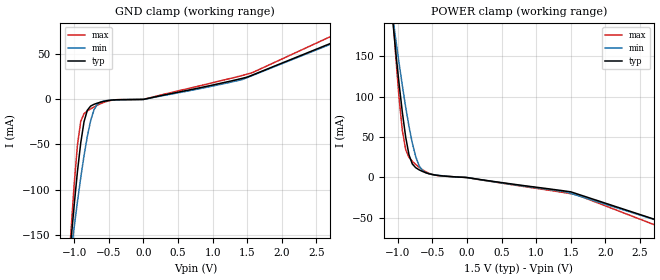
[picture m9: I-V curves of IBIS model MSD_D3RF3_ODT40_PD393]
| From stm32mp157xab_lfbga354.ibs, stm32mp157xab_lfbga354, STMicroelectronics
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[Model] MSD_D3RF3_ODT40_PD393
Model_type   Input
C_comp 2.254pF   2.214pF   2.330pF
Vinh = 925.000mV
Vinl = 575.000mV
[Model Spec]
Vinh   925.000mV   888.000mV   963.000mV
Vinl   575.000mV   538.000mV   613.000mV
[Temperature Range]   25.000   125.000   -40.000
[Voltage Range]   1.500V   1.425V   1.575V
[GND Clamp Reference]   0.00V   0.00V   0.00V
[POWER Clamp Reference]   1.500V   1.425V   1.575V
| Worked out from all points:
|   GND clamp passes 1 mA (typ) near -0.49 V on its own axis
|   POWER clamp passes 1 mA (typ) near -0.21 V on its own axis
[GND Clamp]
-1.48V    -589mA     -456.8mA   -787.9mA
-1.05V    -159mA     -171.5mA   -149.1mA
-1.002V   -117.6mA   -142mA     -94.67mA
-954.6mV  -80.28mA   -113.7mA   -50.75mA
-906.8mV  -48.39mA   -86.94mA   -24.46mA
-859.1mV  -24.71mA   -62.42mA   -15.81mA
-763.6mV  -7.4mA     -23.69mA   -10.51mA
-715.9mV  -5.48mA    -11.75mA   -8.46mA
-620.5mV  -3.1mA     -2.84mA    -4.812mA
900nV     15.27nA    13.81nA    17.99nA
1.575V    27mA       26.51mA    29.69mA
2.959V    69.98mA    68.96mA    78.7mA
[Power Clamp]
-1.459V   582.4mA    458.3mA    771.6mA
-1.077V   197.4mA    201.1mA    207.6mA
-1.03V    155mA      170.7mA    149.6mA
-981.8mV  115.7mA    141.2mA    97.87mA
-934.1mV  80.12mA    113.1mA    57.63mA
-886.4mV  49.8mA     86.89mA    34.39mA
-838.6mV  27.94mA    63.1mA     24.86mA
-743.2mV  12.23mA    26.17mA    16.18mA
-647.7mV  7.632mA    9.012mA    9.818mA
-552.3mV  4.676mA    4.712mA    5.325mA
1.548V    -19.06mA   -20.93mA   -20.65mA
2.98V     -59.26mA   -59.33mA   -67.41mA
